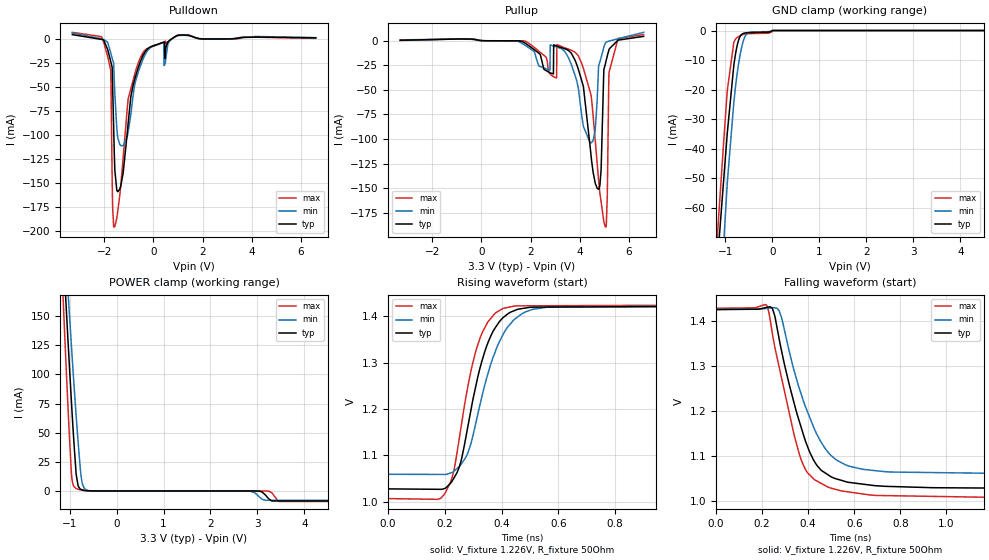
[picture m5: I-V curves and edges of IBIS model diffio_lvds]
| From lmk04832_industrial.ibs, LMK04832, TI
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|   diffio_lvds Model
[Model]   diffio_lvds
Model_type   I/O
Polarity   Non-Inverting
Enable   Active-High
Vinl = 0.4
Vinh = 1.2
Vmeas = 1.226
Vref = 1.226
Cref = 1pF
Rref = 50
|   typ   min   max
C_comp   1.62pF   1.576pF   1.674pF
|  Where Nom  PVT is Nominal Process,   3.3V,  25C
|   Fast PVT is Strong Process,   3.45V, -40C
|   Slow PVT is Weak Process,   3.15V, 85C
[Model spec]
|subparameter
Vinl   0.400   0.370   0.430
Vinh   1.200   1.170   1.230
[Voltage Range]   3.3   3.15   3.45
|Junction Temperature
[Temperature Range]   25   85   -40
[Pullup Reference]   3.3   3.15   3.45
[Pulldown Reference]   0   0   0
[Power Clamp Reference]   3.3   3.15   3.45
[GND Clamp Reference]   0   0   0
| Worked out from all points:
|   slope of the pullup table from 0 to 0.495 V, typ, clamps not added: 2.85 kohm
|   GND clamp passes 1 mA (typ) near -0.62 V on its own axis
|   POWER clamp passes 1 mA (typ) near -0.74 V on its own axis
|   falling waveform, V_fixture 1.226V, R_fixture 50Ohm: 20-80 % time 129ps typ, 145ps min, 116ps max; typ from 1.43 V to 1.03 V
|   rising waveform, V_fixture 1.226V, R_fixture 50Ohm: 20-80 % time 88.5ps typ, 102ps min, 78.9ps max; typ from 1.03 V to 1.42 V
[Pulldown]
|   Voltage   I(typ)   I(min)   I(max)
-3.3V     4.552mA    6.192mA    6.962mA
-2.11V    -437.5uA   325.8uA    2.461mA
-1.74V    -23.23mA   -14.21mA   -32.29mA
-1.66V    -50.24mA   -21.9mA    -175.5mA
-1.6V     -112.1mA   -38.66mA   -196.1mA
-1.49V    -157.7mA   -93.78mA   -186.5mA
-1.24V    -140.7mA   -111.3mA   -125.7mA
-1.03V    -87.91mA   -97.1mA    -62.62mA
-770mV    -42.78mA   -48.54mA   -37.48mA
-350mV    -13.81mA   -16.87mA   -11.7mA
1V        3.854mA    3.519mA    4.175mA
6.6V      1.269mA    1.361mA    703.8uA
[GND Clamp]
|   Voltage   I(typ)   I(min)   I(max)
-3.3V     -880.2mA   -824.9mA   -955.5mA
-1.18V    -80.5mA    -122.1mA   -71.85mA
-1.04V    -51.39mA   -73.25mA   -38.58mA
-960mV    -34.84mA   -51.71mA   -20.4mA
-820mV    -11.74mA   -24.32mA   -3.983mA
-730mV    -3.862mA   -12.43mA   -2.166mA
-670mV    -1.608mA   -6.896mA   -1.634mA
-620mV    -991.5uA   -3.63mA    -1.335mA
-570mV    -794.2uA   -1.677mA   -1.162mA
-500mV    -706.1uA   -676.8uA   -1.062mA
0V        0A         0A         0A
6.6V      0A         0A         0A
[Pullup]
|   Voltage   I(typ)   I(min)   I(max)
-3.3V     609.8uA    1.015mA    385.9uA
3.06V     -5.171mA   -6.237mA   -37.83mA
3.83V     -21.01mA   -36.7mA    -12.05mA
4.44V     -112.1mA   -104.1mA   -53.32mA
4.63V     -145mA     -91.39mA   -101.4mA
4.76V     -151.2mA   -29.79mA   -139.8mA
4.87V     -131mA     -16.94mA   -164.1mA
4.98V     -29.49mA   -6.503mA   -184mA
5.06V     -21.56mA   -1.674mA   -189.8mA
5.12V     -15.43mA   -822.3uA   -158.6mA
5.19V     -9.038mA   -252.1uA   -32.36mA
6.6V      4.581mA    8.703mA    6.43mA
[POWER Clamp]
|   Voltage   I(typ)   I(min)   I(max)
-3.3V     1.944A     1.741A     2.257A
-1.23V    279.5mA    301.8mA    251.5mA
-1.11V    186.9mA    221.6mA    140.1mA
-1.07V    156.6mA    195.3mA    104.1mA
-1.01V    112.1mA    156.2mA    52.47mA
-960mV    76.51mA    124.5mA    14.98mA
-920mV    49.82mA    99.77mA    4.868mA
-860mV    14.5mA     64.71mA    2.062mA
-820mV    4.859mA    43.26mA    1.488mA
-740mV    963.9uA    8.663mA    758.6uA
-610mV    149uA      399.9uA    139uA
6.6V      -8.594mA   -8.021mA   -9.078mA
[Ramp]
R_load = 50
|   typ   min   max
dV/dt_r   0.237282/8.83338e-11   0.218767/1.01327e-10   0.251489/7.8619e-11
dV/dt_f   0.23773/1.28618e-10   0.219171/1.45022e-10   0.25194/1.15754e-10
[Falling Waveform]
V_fixture = 1.226V
V_fixture_min = 1.242V
V_fixture_max = 1.217V
R_fixture = 50Ohm
C_fixture = 0F
|   Time   V(typ)   V(min)   V(max)
0s        1.425V     1.425V     1.428V
213ps     1.429V     1.427V     1.436V
242.3ps   1.429V     1.429V     1.379V
284.3ps   1.334V     1.408V     1.274V
341.6ps   1.213V     1.285V     1.142V
392.8ps   1.127V     1.204V     1.067V
440.3ps   1.078V     1.146V     1.044V
497.3ps   1.055V     1.103V     1.03V
669.2ps   1.036V     1.069V     1.014V
10ns      1.028V     1.06V      1.008V
[Rising Waveform]
V_fixture = 1.226V
V_fixture_min = 1.242V
V_fixture_max = 1.217V
R_fixture = 50Ohm
C_fixture = 0F
|   Time   V(typ)   V(min)   V(max)
0s        1.028V     1.059V     1.007V
176.5ps   1.027V     1.059V     1.005V
224.9ps   1.044V     1.063V     1.051V
255.8ps   1.085V     1.08V      1.156V
282.3ps   1.166V     1.107V     1.253V
323.2ps   1.287V     1.208V     1.352V
386.5ps   1.384V     1.338V     1.411V
446.5ps   1.413V     1.394V     1.423V
581.1ps   1.42V      1.421V     1.423V
10ns      1.423V     1.424V     1.426V
